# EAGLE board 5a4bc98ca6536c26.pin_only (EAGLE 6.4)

Size 15.24 x 15.24 mm. Coordinates in mm from the lower left corner, seen from the top.
Outline: 0,0 15.22,0 15.24,15.24 0,15.24 0,0
Copper layers (1*16): Top 0.035mm / dielectric 1.5mm / Bottom 0.035mm
Design rules "SparkFun *": minimum track width 7mil, minimum drill 15mil, track to track 8mil, track to pad 8mil, pad to pad 8mil, via to via 8mil, smd to smd 8mil, copper to edge 8mil, drill to drill 8mil, minimum pad ring 12mil, minimum via ring 10mil, stop-mask expansion 4mil, vias tented up to drill 20mil, thermal gap 10mil

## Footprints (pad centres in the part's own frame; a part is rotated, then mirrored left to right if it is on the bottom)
0603-CAP = smd 1.1 x 1: 1 -0.85,0; 2 0.85,0
EIA3216 = smd 1.4 x 1.6: A 1.4,0; C -1.4,0
MICRO-FIDUCIAL = smd 0.635 x 0.635: 1 0,0
1X05_ROUNDONLY_NOSILK = drill 1.016 pad 1.88: 1 0,0; 2 2.54,0; 3 5.08,0; 4 7.62,0; 5 10.16,0
0603-RES = smd 1.1 x 1: 1 -0.85,0; 2 0.85,0
SJ_3_PASTE1&2&3 = smd 0.635 x 1.27: 1 -0.813,0; 2 0,0; 3 0.813,0
SJ_2S = smd 0.635 x 1.27: 1 -0.412,0; 2 0.412,0
STAND-OFF = hole 3.302: 0,0
BMP180 = smd 0.6 x 0.5: 1 1.5,1.45; 2 0,1.45; 3 -1.5,1.45; 4 -1.5,-1.45; 5 0,-1.45; 6 1.5,-1.45 | smd 0.5 x 0.6: 7 1.5,0

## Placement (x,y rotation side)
C1  0.1uF  [0603-CAP]  7.62,11.11 0 top
C2  0.1uF  [0603-CAP]  3.81,5.08 270 top
C3  10uF  [EIA3216]  2.54,8.26 0 top
FID1  FIDUCIALUFIDUCIAL  [MICRO-FIDUCIAL]  14.29,10.79 0 top
FID2  FIDUCIALUFIDUCIAL  [MICRO-FIDUCIAL]  0.95,2.54 0 top
FRAME1  FRAME-LETTER  [CREATIVE_COMMONS]  not placed on the board
JP1  [1X05_ROUNDONLY_NOSILK]  2.54,1.27 0 top
LOGO1  LOGO-SFENW2  [SFE-NEW-WEB]  13.97,7.94 0 bottom
LOGO2  OSHW-LOGOS  [OSHW-LOGO-S]  7.62,7.14 0 bottom
R1  4.7K  [0603-RES]  13.97,5.08 90 top
R2  4.7K  [0603-RES]  11.43,5.08 90 top
SJ1  [SJ_3_PASTE1&2&3]  12.7,8.26 0 top
SJ2  [SJ_2S]  1.27,4.6 0 top
STANDOFF1  STAND-OFF  [STAND-OFF]  12.7,12.7 0 top
STANDOFF2  STAND-OFF  [STAND-OFF]  2.54,12.7 0 top
U1  BMP180  [BMP180]  7.62,7.62 0 top

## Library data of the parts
C1 C2 = SparkFun-Capacitors
C3 = SparkFun-Capacitors; PROD_ID: CAP-00811
FID1 FID2 FRAME1 LOGO1 LOGO2 = SparkFun-Aesthetics
JP1 SJ1 SJ2 = mike-temp
R1 R2 = SparkFun-Passives
STANDOFF1 STANDOFF2 = SparkFun-Electromechanical
U1 = SparkFun-Sensors

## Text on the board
Bottom: V10
tPlace: BMP180 | BARO | SJ1 | SJ2 | IO | + | - | CL | DA
bPlace: BMP180 | BARO | VDDIO | VDD | GND | SCL | SDA
tValues: M Grusin
Measures: 0.125 X 2

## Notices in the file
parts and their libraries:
SparkFun-Aesthetics: Licensing: CC v3.0 Share-Alike You are welcome to use this library for commercial purposes.
SparkFun-Aesthetics: Released under the Creative Commons Attribution Share-Alike 3.0 License
SparkFun-Aesthetics: http://creativecommons.org/licenses/by-sa/3.0
